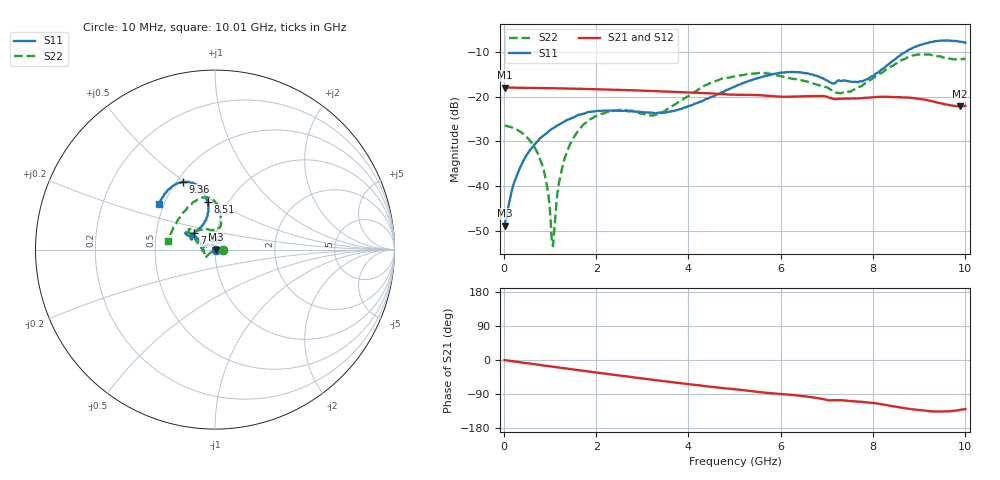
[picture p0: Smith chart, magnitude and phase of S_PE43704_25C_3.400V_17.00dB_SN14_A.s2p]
! Device ID: PE43704
! Dir: z:\PE43704\PE43704_Char_1_20130516\PE43704\AMB\3p400V\17p00dB
! Serial: 14
! Insertion: A
! Impedance: 50 ohm
! Temp: Amb
! VDD: 3.400V
! Attenuation Step: 17.00dB
! IDD: 1.139999e-01mA
#  Hz  S  RI  R  50
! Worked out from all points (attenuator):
!   401 points, 10 MHz to 10.01 GHz, reference 50 ohm
!   highest |S21| = -17.96 dB at 10 MHz (marker M1); lowest = -22.2 dB at 9.885 GHz (marker M2)
!   lowest |S11| = -48.8 dB at 10 MHz (marker M3), VSWR 1.01, Z = 50.4 + j0.0458 ohm
!   |S11| at or under -10 dB: start of sweep to 8.713 GHz
!   |S22| runs from -53.5 to -10.5 dB; largest |S21 - S12| = 0.0012
!   S11 on the Smith chart (normalised r, x): 10 MHz: 1.01, +0.00; 7.46 GHz: 0.78, +0.15; 8.51 GHz: 0.81, +0.46; 9.36 GHz: 0.54, +0.49; 10.01 GHz: 0.47, +0.28
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1e7  0.00358 0.000455  0.1265 -0.000468  0.1265 -0.000341  0.0471 -3.02e-05
2.85e8  0.00102 0.0135  0.1254 -0.0108  0.1254 -0.0108  0.0423 0.00421
7.1e8  -0.014 0.0277  0.1223 -0.026  0.1223 -0.026  0.0238 0.00553
9.1e8  -0.0246 0.0297  0.1201 -0.0329  0.1201 -0.0328  0.011 0.00225
1.01e9  -0.0303 0.0302  0.1189 -0.0362  0.119 -0.0361  0.00406 -6.59e-05
1.06e9  -0.033 0.0295  0.1183 -0.038  0.1184 -0.0379  0.000434 -0.00208
1.185e9  -0.0395 0.028  0.1165 -0.0421  0.1165 -0.042  -0.00826 -0.00651
1.285e9  -0.0446 0.0264  0.1149 -0.0452  0.1149 -0.0452  -0.0152 -0.0102
1.685e9  -0.0617 0.015  0.108 -0.0574  0.1079 -0.0573  -0.0374 -0.0277
2.36e9  -0.0696 -0.00396  0.0933 -0.0749  0.0934 -0.0748  -0.0542 -0.0429
3.36e9  -0.0664 -0.001  0.0672 -0.0933  0.0673 -0.0932  -0.0634 -0.00737
4.41e9  -0.0842 0.043  0.0382 -0.1025  0.0384 -0.1024  -0.1172 0.0701
5.01e9  -0.1085 0.0714  0.0232 -0.1027  0.0232 -0.1028  -0.1416 0.0921
5.96e9  -0.1569 0.0954  0.00116 -0.1002  0.00176 -0.1002  -0.1332 0.1074
6.685e9  -0.157 0.0821  -0.015 -0.1005  -0.0148 -0.1004  -0.0924 0.1075
7.46e9  -0.1151 0.0941  -0.0291 -0.0906  -0.0292 -0.0908  0.00592 0.1135
7.835e9  -0.0688 0.138  -0.0354 -0.0902  -0.0353 -0.0901  0.0317 0.137
8.36e9  -0.0369 0.2308  -0.0502 -0.0856  -0.0502 -0.0862  0.0277 0.2084
8.51e9  -0.0397 0.2658  -0.0544 -0.0824  -0.0541 -0.083  0.0187 0.2351
9.36e9  -0.1786 0.378  -0.0624 -0.0605  -0.0626 -0.0607  -0.1243 0.2624
9.885e9  -0.2926 0.2914  -0.0522 -0.058  -0.0522 -0.058  -0.2395 0.1028
1.001e10  -0.3119 0.2532  -0.0503 -0.0611  -0.0512 -0.0614  -0.2607 0.0507
